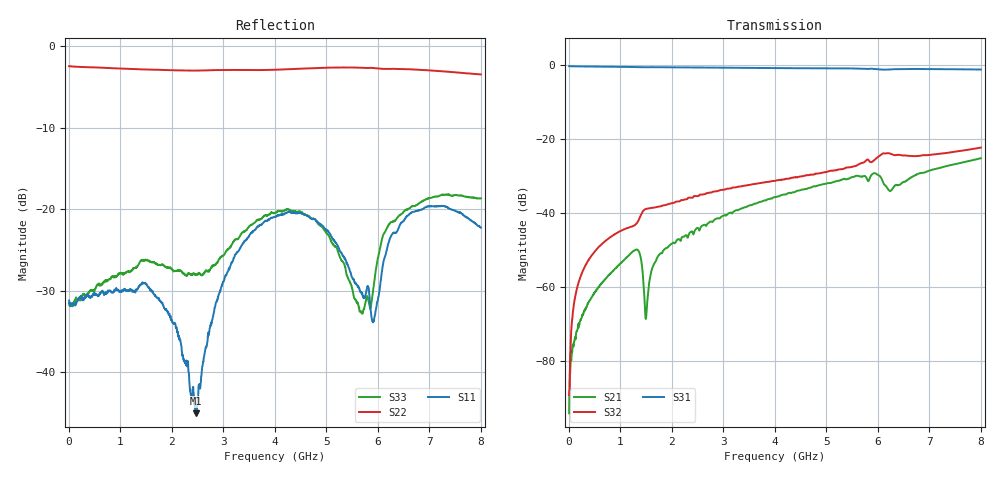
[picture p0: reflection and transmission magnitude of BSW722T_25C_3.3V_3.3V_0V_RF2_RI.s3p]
! Product: BSW722T
! Temp: 25C
! VDD: 3.300
! Control_Hi: 3.300
! Control_Lo: 0.000
! Logic State: RF2
! Port 1: RFC
! Port 2: RF1
! Port 3: RF2
! V1 = 0.00
! V2 = 0.00
! V3 = 0.00
! V4 = 0.00
# Hz S  RI  R 50
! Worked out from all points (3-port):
!   1601 points, 5 MHz to 8.005 GHz, reference 50 ohm
!   strongest paths, dB at 5 MHz, 2.005 GHz, 4.005 GHz, 6.005 GHz, 8.005 GHz:
!     S31: -0.3, -0.6, -0.8, -1.1, -1.2
!     S32: -89.2, -37.3, -31.3, -24.9, -22.3
!     S21: -94.1, -48.3, -35.7, -29.7, -25.2
!   lowest |S11| = -45.0 dB at 2.465 GHz (marker M1), VSWR 1.01, Z = 49.5 + j0.297 ohm
!   |S11| at or under -10 dB: start of sweep to end of sweep
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5000000  0.0275 -0.00172  -1.2e-06 -6.94e-06  0.9672 -0.01
         1.41e-07 -1.96e-05  -0.7547 0.00734  -3.53e-06 3.49e-05
         0.9672 -0.0098  1.12e-06 3.45e-05  0.0267 -0.000924
2.8e8  0.0238 -0.015  -7.5e-05 0.00043  0.8596 -0.4246
       -7.49e-05 0.000418  -0.6725 0.322  0.000648 0.00158
       0.8596 -0.4245  0.000631 0.00158  0.0256 -0.0157
1.08e9  -0.0223 -0.023  0.00225 0.000666  -0.1703 -0.9303
        0.00225 0.000685  0.0963 0.7221  0.00604 0.000365
        -0.1706 -0.9304  0.00606 0.000362  -0.0237 -0.0331
1.505e9  -0.0346 0.00438  0.000416 -9.81e-05  -0.7101 -0.6107
         0.000404 -8.46e-05  0.5184 0.5007  0.0103 -0.00499
         -0.7098 -0.6104  0.0103 -0.00499  -0.0477 -0.00932
2.465e9  -0.00475 0.003  0.00212 -0.00567  -0.6253 0.6862
         0.00211 -0.00567  0.4958 -0.5074  -0.00694 -0.0155
         -0.6255 0.6862  -0.00697 -0.0155  -0.0291 0.0267
4.005e9  0.0258 0.0861  -0.0136 0.00924  0.9004 -0.1443
         -0.0136 0.00928  -0.697 0.1714  -0.0125 0.0242
         0.9008 -0.1445  -0.0125 0.0242  0.0401 0.0858
4.92e9  0.0761 -0.0233  0.0127 0.0209  -0.0483 -0.9047
        0.0127 0.0209  0.0527 0.7357  0.0251 0.0244
        -0.0481 -0.9043  0.0251 0.0244  0.075 -0.0216
5.865e9  -0.0236 0.00409  0.0262 -0.0178  -0.8948 0.00701
         0.0262 -0.0178  0.7301 0.1003  0.0404 -0.0274
         -0.8946 0.00664  0.0404 -0.0273  -0.0191 0.017
6.9e9  0.1014 0.00737  -0.0151 -0.0318  0.0818 0.8809
       -0.0151 -0.0317  0.1302 -0.7023  -0.0412 -0.0444
       0.0814 0.8804  -0.0412 -0.0445  0.1127 0.0125
8.005e9  -0.0629 -0.0447  -0.0402 0.0377  0.8255 -0.2796
         -0.0402 0.0378  -0.6703 0.0487  -0.0552 0.0536
         0.8254 -0.2793  -0.0552 0.0535  0.0527 -0.1043
